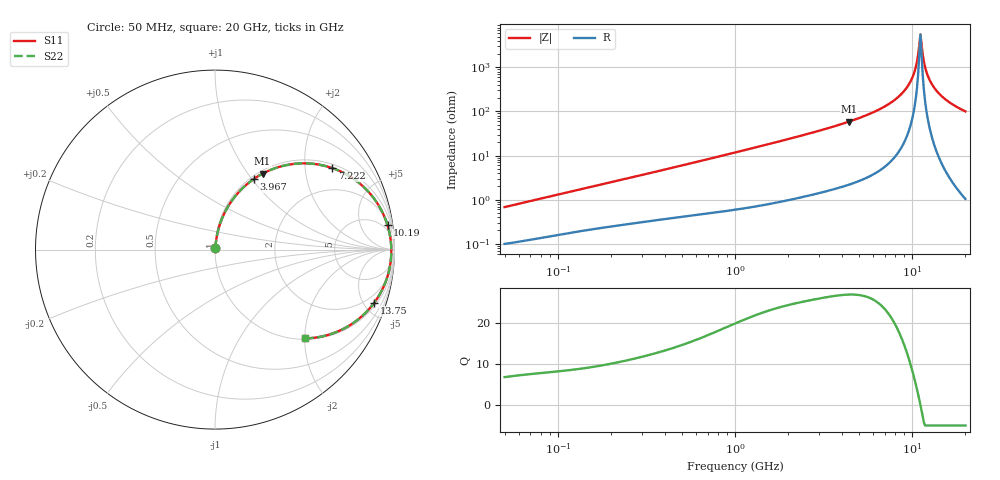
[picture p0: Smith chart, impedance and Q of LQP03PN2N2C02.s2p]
!Murata Part Number: LQP03PN2N2C02
!These Parameters are Measured in Series Mode Connection
!  o--[Z]--o
!Port1  Port2
!  o-------o
!Freq. Start=50[MHz] Stop=20[GHz], 401[Steps]
# Hz S RI R 50
!Freq.(Hz) S11(Real) S11(Imag) S21(Real) S21(Imag) S12(Real) S12(Imag) S22(Real) S22(Imag)
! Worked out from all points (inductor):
!   401 points, 50 MHz to 20 GHz, reference 50 ohm
!   read as one part in series: L = 2.11 nH near 51.52 MHz
!   highest Q = 26.9 at 4.406 GHz (marker M1), where L = 2.13 nH
!   self-resonance near 10.99 GHz
!   S11 on the Smith chart (normalised r, x): 50 MHz: 1.00, +0.01; 3.967 GHz: 1.04, +1.03; 7.222 GHz: 1.12, +2.79; 10.19 GHz: 3, +14; 13.75 GHz: 1.24, -5.87; 20 GHz: 1.02, -2.01
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5e7  0.00104 0.0067  0.999 -0.0067  0.999 -0.0067  0.00104 0.0067
1.364002e8  0.00225 0.0172  0.9978 -0.0172  0.9978 -0.0172  0.00225 0.0172
3.721004e8  0.00544 0.0443  0.9946 -0.0443  0.9946 -0.0443  0.00544 0.0443
1e9  0.0192 0.1142  0.9808 -0.1142  0.9808 -0.1142  0.0192 0.1142
2.728004e9  0.1076 0.2909  0.8924 -0.2909  0.8924 -0.2909  0.1076 0.2909
3.967106e9  0.2172 0.394  0.7828 -0.394  0.7828 -0.394  0.2172 0.394
4.405649e9  0.2652 0.4232  0.7348 -0.4232  0.7348 -0.4232  0.2652 0.4232
7.222371e9  0.6538 0.4542  0.3462 -0.4542  0.3462 -0.4542  0.6538 0.4542
7.442007e9  0.6854 0.4421  0.3146 -0.4421  0.3146 -0.4421  0.6854 0.4421
9.041845e9  0.881 0.2911  0.119 -0.2911  0.119 -0.2911  0.881 0.2911
9.745021e9  0.9372 0.1985  0.0628 -0.1985  0.0628 -0.1985  0.9372 0.1985
1.019291e10  0.9613 0.1355  0.0387 -0.1355  0.0387 -0.1355  0.9613 0.1355
1.050288e10  0.9726 0.0911  0.0274 -0.0911  0.0274 -0.0911  0.9726 0.0911
1.082228e10  0.9796 0.0456  0.0204 -0.0456  0.0204 -0.0456  0.9796 0.0456
1.115139e10  0.9824 -0.000708  0.0176 0.000708  0.0176 0.000708  0.9824 -0.000708
1.131968e10  0.9821 -0.0239  0.0179 0.0239  0.0179 0.0239  0.9821 -0.0239
1.183995e10  0.9747 -0.093  0.0253 0.093  0.0253 0.093  0.9747 -0.093
1.220001e10  0.9644 -0.1379  0.0356 0.1379  0.0356 0.1379  0.9644 -0.1379
1.276073e10  0.9414 -0.2022  0.0586 0.2022  0.0586 0.2022  0.9414 -0.2022
1.375312e10  0.8862 -0.2974  0.1138 0.2974  0.1138 0.2974  0.8862 -0.2974
1.621653e10  0.7201 -0.4392  0.2799 0.4392  0.2799 0.4392  0.7201 -0.4392
2e10  0.5023 -0.4948  0.4977 0.4948  0.4977 0.4948  0.5023 -0.4948
